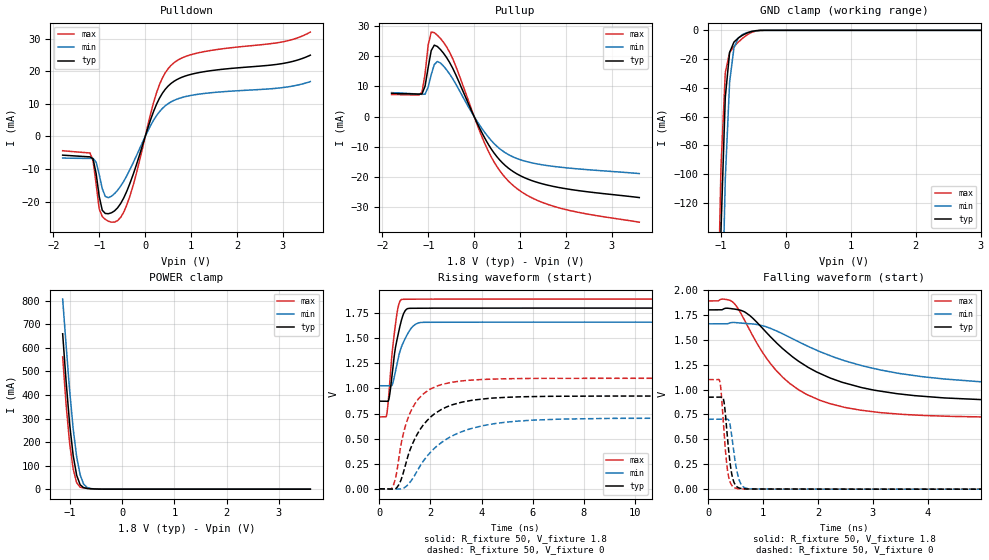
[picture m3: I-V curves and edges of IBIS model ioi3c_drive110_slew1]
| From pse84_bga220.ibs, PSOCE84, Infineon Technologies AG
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[Model] ioi3c_drive110_slew1
Model_type I/O
Enable   Active-High
Vinl  =  0.54
Vinh  =  1.26
Vmeas =  0.9
Cref  =  15e-12
| Capacitance   typ   min   max
C_comp   9.12545e-13 8.87504e-13 9.42456e-13
| Variables   typ   min   max
[GND Clamp Reference]   0   0   0
[POWER Clamp Reference]   1.8   1.66   1.89
[Pulldown Reference]   0   0   0
[Pullup Reference]   1.8   1.66   1.89
[Temperature Range]   25   125   -40
[Voltage Range]   1.8   1.66   1.89
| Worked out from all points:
|   slope of the pulldown table from 0 to 0.27 V, typ, clamps not added: 25.6 ohm
|   slope of the pullup table from 0 to 0.27 V, typ, clamps not added: 33.1 ohm
|   GND clamp passes 1 mA (typ) near -0.55 V on its own axis
|   POWER clamp passes 1 mA (typ) near -0.54 V on its own axis
|   falling waveform, R_fixture 50, V_fixture 1.8: 20-80 % time 1.55ns typ, 2.14ns min, 1.09ns max; typ from 1.8 V to 0.873 V
|   falling waveform, R_fixture 50, V_fixture 0: 20-80 % time 103ps typ, 117ps min, 95.1ps max; typ from 0.923 V to 0 V
|   rising waveform, R_fixture 50, V_fixture 1.8: 20-80 % time 335ps typ, 467ps min, 262ps max; typ from 0.873 V to 1.8 V
|   rising waveform, R_fixture 50, V_fixture 0: 20-80 % time 1.15ns typ, 1.75ns min, 768ps max; typ from 0 V to 0.923 V
[GND Clamp]
| Voltage   I(typ)   I(min)   I(max)
-1.204V   -737.9mA   -831.5mA   -678.7mA
-1.07V    -303.2mA   -410.8mA   -239.8mA
-1.003V   -139.9mA   -232.2mA   -95.74mA
-936.6mV  -46.51mA   -103.5mA   -29.5mA
-869.7mV  -15.31mA   -35.88mA   -15.36mA
-802.8mV  -8.166mA   -12.13mA   -11.29mA
-735.9mV  -5.335mA   -5.292mA   -8.195mA
-669mV    -3.356mA   -2.85mA    -5.457mA
-535.2mV  -837.9uA   -772uA     -1.483mA
-401.4mV  -47.36uA   -84.85uA   -76.77uA
3.6V      0A         0A         0A
[POWER Clamp]
| Voltage   I(typ)   I(min)   I(max)
-1.137V   660mA      807.5mA    561.8mA
-1.07V    454.5mA    608.2mA    356.2mA
-1.003V   275.7mA    418.4mA    193.6mA
-936.6mV  143.5mA    257.2mA    86.91mA
-869.7mV  59.43mA    137.9mA    27.31mA
-802.8mV  18.8mA     60.93mA    8.704mA
-735.9mV  6.231mA    21.35mA    5.155mA
-669mV    3.127mA    6.887mA    3.44mA
-535.2mV  940.9uA    1.232mA    1.058mA
-334.5mV  16.1uA     59.03uA    7.686uA
3.6V      0A         0A         0A
[Pulldown]
| Voltage   I(typ)   I(min)   I(max)
-1.8V     -5.733mA   -6.614mA   -4.376mA
-1.204V   -6.26mA    -6.73mA    -5.062mA
-1.137V   -6.869mA   -6.73mA    -7.434mA
-1.003V   -18.36mA   -11.66mA   -22.25mA
-936.6mV  -22.64mA   -16.01mA   -24.56mA
-869.7mV  -23.63mA   -18.41mA   -25.45mA
-669mV    -22.83mA   -17.54mA   -26.27mA
-401.4mV  -16.78mA   -12.04mA   -21.01mA
248.3mV   9.926mA    6.426mA    13.46mA
558.6mV   16.21mA    10.57mA    21.74mA
1.117V    19.44mA    12.87mA    25.53mA
3.6V      24.94mA    16.84mA    32.02mA
[Pullup]
| Voltage   I(typ)   I(min)   I(max)
-1.8V     7.687mA    7.955mA    7.314mA
-1.137V   7.536mA    7.382mA    8.126mA
-1.07V    10.11mA    7.436mA    14.18mA
-1.003V   16.28mA    9.774mA    23.7mA
-936.6mV  21.89mA    13.9mA     28.01mA
-869.7mV  23.68mA    17.26mA    27.82mA
-735.9mV  22.24mA    17.77mA    25.91mA
-468.3mV  16.03mA    12.55mA    19.19mA
310.3mV   -9.225mA   -6.811mA   -11.53mA
806.9mV   -17.76mA   -13.06mA   -22.23mA
1.738V    -23.16mA   -16.51mA   -29.74mA
3.6V      -26.82mA   -18.88mA   -34.98mA
[Ramp]
dV/dt_r   0.554053/1.15235n  0.421104/1.74923n  0.660024/0.767532n
dV/dt_f   0.556218/1.54811n  0.379912/2.13555n  0.704096/1.0927n
R_load = 50
[Falling Waveform]
R_fixture = 50
V_fixture = 1.8
V_fixture_min = 1.66
V_fixture_max = 1.89
| Time   V(typ)   V(min)   V(max)
0s        1.8V       1.66V      1.89V
459.4ps   1.81V      1.674V     1.873V
746.6ps   1.749V     1.661V     1.608V
1.23ns    1.477V     1.593V     1.197V
1.65ns    1.284V     1.479V     997.2mV
2.203ns   1.121V     1.345V     860.8mV
3.042ns   992.3mV    1.209V     775.2mV
3.895ns   933.5mV    1.13V      740.8mV
6.553ns   880.5mV    1.046V     717.3mV
800ns     873mV      1.027V     716.5mV
[Falling Waveform]
R_fixture = 50
V_fixture = 0
V_fixture_min = 0
V_fixture_max = 0
| Time   V(typ)   V(min)   V(max)
0s        923.4mV    701.8mV    1.1V
213.5ps   923.2mV    701.8mV    1.078V
241.7ps   924mV      701.8mV    940.8mV
290.4ps   868.9mV    701.7mV    553.2mV
349.2ps   527.2mV    703mV      200.8mV
414.5ps   201.1mV    594.7mV    52.07mV
508.7ps   31.99mV    222.4mV    8.961mV
593.7ps   7.135mV    54.72mV    2.855mV
1.01ns    1.221mV    1.197mV    794.4uV
800ns     9.104nV    625.7nV    3.374nV
[Rising Waveform]
R_fixture = 50
V_fixture = 1.8
V_fixture_min = 1.66
V_fixture_max = 1.89
| Time   V(typ)   V(min)   V(max)
0s        873mV      1.027V     716.5mV
295ps     873.1mV    1.027V     743.2mV
390.8ps   909mV      1.027V     988.4mV
524.8ps   1.188V     1.049V     1.405V
619.6ps   1.384V     1.152V     1.61V
764.7ps   1.569V     1.325V     1.838V
908.7ps   1.715V     1.44V      1.887V
1.016ns   1.775V     1.498V     1.888V
1.411ns   1.799V     1.639V     1.889V
800ns     1.8V       1.66V      1.89V
[Rising Waveform]
R_fixture = 50
V_fixture = 0
V_fixture_min = 0
V_fixture_max = 0
| Time   V(typ)   V(min)   V(max)
0s        9.105nV    625.5nV    3.376nV
550.2ps   -3.136mV   -1.542mV   34.01mV
793.4ps   54.13mV    -2.241mV   351.4mV
1.007ns   222.1mV    15.58mV    612mV
1.528ns   562.5mV    197.3mV    894.7mV
2.186ns   751.8mV    410mV      1.016V
3.442ns   873.2mV    588.5mV    1.08V
5.325ns   914.6mV    672.7mV    1.098V
9.095ns   924.1mV    701.7mV    1.101V
50ns      923.4mV    701.8mV    1.1V
